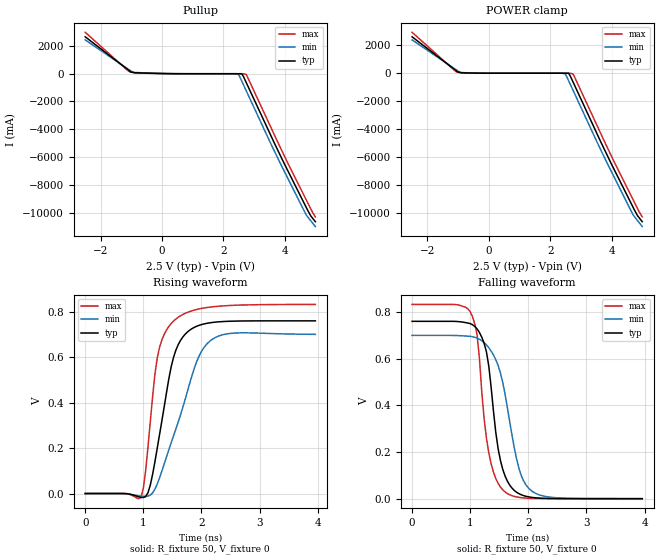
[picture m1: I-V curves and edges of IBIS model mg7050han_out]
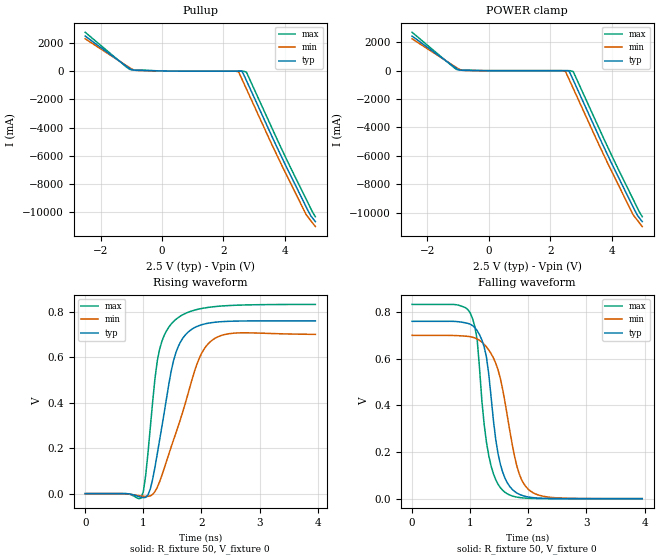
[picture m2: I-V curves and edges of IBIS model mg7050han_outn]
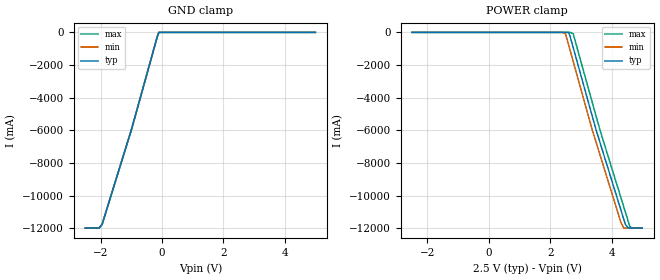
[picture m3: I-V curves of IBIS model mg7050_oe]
|   IBIS File mg7050han_4a_25v_100.ibs  ZSEL=H(ZO=100ohm)
[IBIS Ver]   3.2
[Comment Char]   |_char
[File name]   mg7050han_4a_25v_100.ibs
[File Rev]   1.0
[Date]   Jan 23, 2014
[Source]
|   Component MG7050HAN HCSL 4-OUTPUT 2.5V
[Component]   mg7050han-hcsl-4out-100ohm
[Manufacturer]   Seiko Epson Corporation
[Package]
| variable   typ   min   max
R_pkg   0.27   NA   NA
L_pkg   1.66n   NA   NA
C_pkg   0.53p   NA   NA
[Pin]   signal_name   model_name   R_pin   L_pin   C_pin
1   vcc1   POWER   NA   NA   NA
2   out1p   mg7050han_out   0.34   2.1nH   0.58pF
3   out1n   mg7050han_outn  0.25   1.5nH   0.50pF
4   out2p   mg7050han_out   0.22   1.3nH   0.44pF
5   out2n   mg7050han_outn  0.25   1.7nH   0.59pF
6   zsel   mg7050_zsel   NA   NA   NA
7   oe   mg7050_oe   NA   NA   NA
8   out3n   mg7050han_outn  0.25   1.7nH   0.62pF
9   out3p   mg7050han_out   0.22   1.3nH   0.49pF
10   out4n   mg7050han_outn  0.25   1.5nH   0.46pF
11   out4p   mg7050han_out   0.34   2.1nH   0.57pF
12   vcc2   POWER   NA   NA   NA
13   vcc   POWER   NA   NA   NA
14   gnd   GND   NA   NA   NA
[Diff Pin] inv_pin vdiff   tdelay_typ
2   3   0   0
4   5   0   0
9   8   0   0
11   10   0   0
| Models and submodels in the file (4): mg7050han_out (Open_source), mg7050han_outn (Open_source), mg7050_oe (Input), mg7050_zsel (Input)
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[Model]   mg7050han_out
Model_type Open_source
Enable Active-High
Polarity Non-Inverting
Vref=0
Vmeas=0.375
Rref=50
Cref=0
C_comp   5.00p   4.90p   5.21p
[Temperature Range] 25   85   -40
[Voltage Range]   2.5   2.375   2.625
[POWER Clamp Reference]2.5   2.375   2.625
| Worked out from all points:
|   slope of the pullup table from 0 to 0.375 V, typ, clamps not added: 32.3 ohm
|   POWER clamp passes 1 mA (typ) near -0.15 V on its own axis
|   falling waveform, R_fixture 50, V_fixture 0: 20-80 % time 239ps typ, 334ps min, 213ps max; typ from 0.761 V to 0 V
|   rising waveform, R_fixture 50, V_fixture 0: 20-80 % time 323ps typ, 518ps min, 242ps max; typ from 0 V to 0.761 V
[Pullup]
-2.5V     2.638A     2.415A     2.961A
-1.05V    175.8mA    241.6mA    116.8mA
-900mV    57.47mA    57.93mA    77.53mA
-750mV    44.28mA    30.79mA    63.26mA
2.4V      -15.28mA   -14.15mA   -16.79mA
2.5V      -15.29mA   -70.63mA   -16.8mA
2.6V      -15.29mA   -543mA     -16.81mA
2.75V     -662.4mA   -1.255A    -72.5mA
3.8V      -5.62A     -6.192A    -5.049A
4.7V      -9.606A    -10.15A    -9.059A
4.85V     -10.23A    -10.58A    -9.717A
5V        -10.65A    -10.99A    -10.3A
[POWER Clamp]
-2.5V     2.61A      2.388A     2.932A
-1.05V    157.3mA    226mA      89.33mA
-900mV    32.3mA     39.41mA    47.42mA
-750mV    21.7mA     12.79mA    36.77mA
2.4V      -191.7pA   -212.1pA   -181.2pA
2.5V      -202.9pA   -60.77mA   -192.4pA
2.6V      -214.1pA   -533.9mA   -203.6pA
2.75V     -652.5mA   -1.246A    -60.77mA
3.8V      -5.61A     -6.183A    -5.038A
4.7V      -9.596A    -10.14A    -9.048A
4.85V     -10.22A    -10.57A    -9.706A
5V        -10.64A    -10.98A    -10.29A
[Falling Waveform]
R_fixture=50
V_fixture=0
V_fixture_min=0
V_fixture_max=0
0s        761.2mV    700.9mV    833.8mV
1ns       751.4mV    696.6mV    802.4mV
1.12ns    728.1mV    689mV      699.8mV
1.24ns    666.5mV    669.9mV    342.2mV
1.32ns    568.7mV    647.8mV    196.8mV
1.48ns    215.1mV    572.1mV    65.88mV
1.6ns     97.03mV    447.8mV    28.93mV
1.84ns    21.32mV    128.3mV    5.536mV
2.04ns    6.238mV    36.69mV    1.414mV
3.96ns    0V         10.71uV    1.036uV
[Rising Waveform]
R_fixture=50
V_fixture=0
V_fixture_min=0
V_fixture_max=0
0s        0V         939.6nV    0V
960ps     -17.22mV   -11.35mV   -16.48mV
1ns       -17.66mV   -12.28mV   22.6mV
1.08ns    3.496mV    -11.14mV   205.3mV
1.24ns    200.8mV    42.26mV    598.2mV
1.36ns    383.7mV    130.9mV    702.2mV
1.56ns    631.8mV    284.5mV    769.2mV
1.92ns    737.5mV    582.6mV    811.3mV
2.2ns     754.4mV    681.9mV    823.2mV
3.96ns    761.2mV    701.5mV    833.6mV
[Ramp]
R_load=50
dV/dt_r   4.567E-1/3.222E-10   4.205E-1/5.167E-10   5.003E-1/2.395E-10
dV/dt_f   4.567E-1/2.353E-10   4.205E-1/3.313E-10   5.003E-1/2.072E-10
|[End   mg7050han_out
[Model]   mg7050han_outn
Model_type Open_source
Enable Active-High
Polarity Inverting
Vref=0
Vmeas=0.375
Rref=50
Cref=0
C_comp   5.00p   4.90p   5.21p
[Temperature Range] 25   85   -40
[Voltage Range]   2.5   2.375   2.625
[POWER Clamp Reference]2.5   2.375   2.625
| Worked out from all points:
|   slope of the pullup table from 0 to 0.375 V, typ, clamps not added: 32.3 ohm
|   POWER clamp passes 1 mA (typ) near -0.15 V on its own axis
|   falling waveform, R_fixture 50, V_fixture 0: 20-80 % time 237ps typ, 335ps min, 211ps max; typ from 0.761 V to 0 V
|   rising waveform, R_fixture 50, V_fixture 0: 20-80 % time 322ps typ, 514ps min, 240ps max; typ from 0 V to 0.761 V
[Pullup]
-2.5V     2.46A      2.27A      2.73A
-1.05V    164mA      227.2mA    112.9mA
-900mV    57.18mA    56.78mA    77.35mA
-750mV    44.21mA    30.73mA    63.13mA
2.4V      -15.28mA   -14.15mA   -16.79mA
2.5V      -15.29mA   -70.63mA   -16.8mA
2.6V      -15.29mA   -543mA     -16.81mA
2.75V     -662.4mA   -1.255A    -72.5mA
3.8V      -5.62A     -6.192A    -5.049A
4.7V      -9.606A    -10.15A    -9.059A
4.85V     -10.23A    -10.58A    -9.717A
5V        -10.65A    -10.99A    -10.3A
[POWER Clamp]
-2.5V     2.434A     2.246A     2.704A
-1.05V    146.8mA    212.6mA    85.8mA
-900mV    32.11mA    38.56mA    47.28mA
-750mV    21.66mA    12.77mA    36.68mA
2.4V      -191.7pA   -212.1pA   -181.2pA
2.5V      -202.9pA   -60.77mA   -192.4pA
2.6V      -214.1pA   -533.9mA   -203.6pA
2.75V     -652.5mA   -1.246A    -60.77mA
3.8V      -5.61A     -6.183A    -5.038A
4.7V      -9.596A    -10.14A    -9.048A
4.85V     -10.22A    -10.57A    -9.706A
5V        -10.64A    -10.98A    -10.29A
[Falling Waveform]
R_fixture=50
V_fixture=0
V_fixture_min=0
V_fixture_max=0
0s        761.2mV    700.9mV    833.8mV
1ns       748.9mV    695.2mV    797mV
1.12ns    721.1mV    685.3mV    681.4mV
1.24ns    651.8mV    662.9mV    318.9mV
1.32ns    532.8mV    638mV      183.8mV
1.44ns    252.5mV    581mV      81.01mV
1.6ns     87.15mV    412.3mV    27.08mV
1.8ns     24.71mV    142.7mV    6.831mV
2.04ns    5.667mV    32.03mV    1.328mV
3.96ns    0V         9.792uV    1.046uV
[Rising Waveform]
R_fixture=50
V_fixture=0
V_fixture_min=0
V_fixture_max=0
0s        443.5nV    2.919uV    0V
960ps     -16.21mV   -10.53mV   -20.15mV
1.04ns    -16.38mV   -12.42mV   79.13mV
1.12ns    20.57mV    -10.08mV   291.2mV
1.24ns    175.1mV    27.77mV    584.4mV
1.36ns    358.2mV    111.7mV    697.5mV
1.56ns    620.8mV    267mV      767.6mV
1.96ns    740.2mV    595mV      813.3mV
2.2ns     754.1mV    678.8mV    823.1mV
3.96ns    761.2mV    701.6mV    833.6mV
[Ramp]
R_load=50
dV/dt_r   4.567E-1/3.204E-10   4.205E-1/5.130E-10   5.003E-1/2.388E-10
dV/dt_f   4.567E-1/2.360E-10   4.205E-1/3.333E-10   5.003E-1/2.074E-10
|[End   mg7050han_out
[Model]   mg7050_oe
Model_type Input
Vinh=1.75
Vinl=0.75
C_comp   3p   3p   3p
[Temperature Range] 25   85   -40
[Voltage Range]   2.5   2.375   2.625
[POWER Clamp Reference]2.5   2.375   2.625
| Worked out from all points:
|   GND clamp passes 1 mA (typ) near -0.10 V on its own axis
[GND Clamp]
-2.5V     -12A       -12A       -12A
-2.05V    -12A       -12A       -12A
-1.95V    -11.77A    -11.77A    -11.77A
-1V       -6A        -6A        -6A
-150mV    -254mA     -254mA     -254mA
-100mV    -25.23uA   -23.33uA   -29.37uA
5V        24.28uA    24.81uA    25.61uA
[POWER Clamp]
-2.5V     24.28uA    23.63uA    26.96uA
2.4V      -23.29uA   -22.62uA   -25.87uA
2.5V      -24.26uA   -84.67mA   -26.95uA
2.6V      -25.23uA   -761.8mA   -28.02uA
2.75V     -931.1mA   -1.778A    -84.67mA
3.35V     -4.994A    -5.84A     -4.148A
3.5V      -6A        -6.759A    -5.163A
4.3V      -10.86A    -11.62A    -10.1A
4.4V      -11.47A    -12A       -10.71A
4.45V     -11.77A    -12A       -11.01A
4.6V      -12A       -12A       -11.92A
5V        -12A       -12A       -12A
